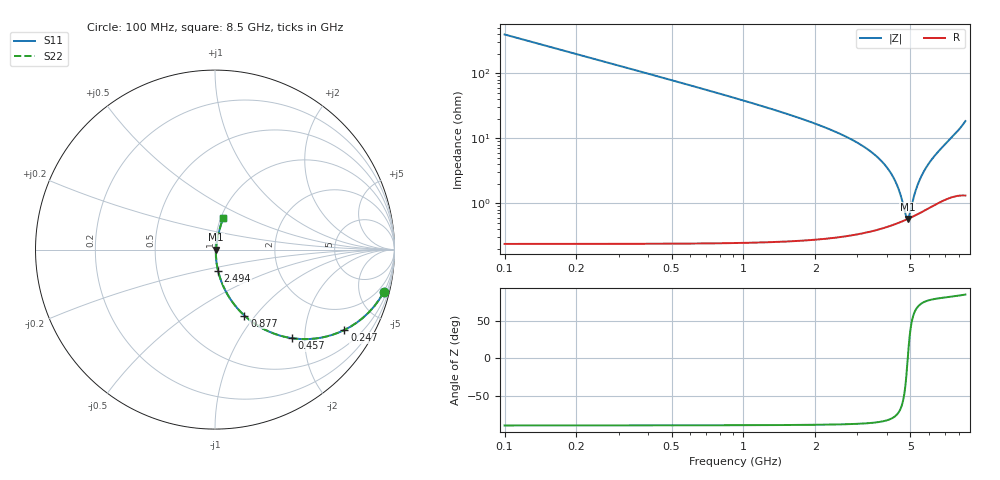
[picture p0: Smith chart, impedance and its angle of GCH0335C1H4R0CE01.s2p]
!Murata Part Number: GCH0335C1H4R0CE01
!These Parameters are Measured in Series Mode Connection
!Data Generated on Mar 13, 2026
!  o--ll--o
!Port1  Port2
!  o------o
!Operation Temp=25[degC], DC Bias Voltage=0[V]
!Freq. Start=100[MHz] Stop=9[GHz] 401[Steps]
# Hz S RI R 50
!Freq.(Hz) S11(Real) S11(Imag) S21(Real) S21(Imag) S12(Real) S12(Imag) S22(Real) S22(Imag)
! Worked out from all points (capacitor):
!   401 points, 100 MHz to 8.5 GHz, reference 50 ohm
!   read as one part in series: C = 4 pF near 142 MHz
!   lowest |Z| = 574 mohm at 4.867 GHz (marker M1)
!   series resonance near 4.875 GHz, so ESL is about 270 pH
!   S11 on the Smith chart (normalised r, x): 100 MHz: 1.00, -7.95; 247 MHz: 1.00, -3.21; 457 MHz: 1.00, -1.73; 877 MHz: 1.00, -0.88; 2.494 GHz: 1.01, -0.24; 8.5 GHz: 1.03, +0.37
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1e8  0.9404 -0.2364  0.0596 0.2364  0.0596 0.2364  0.9404 -0.2364
1.84e8  0.8232 -0.381  0.1768 0.381  0.1768 0.381  0.8232 -0.381
2.47e8  0.7206 -0.448  0.2794 0.448  0.2794 0.448  0.7206 -0.448
3.31e8  0.5888 -0.4911  0.4112 0.4911  0.4112 0.4911  0.5888 -0.4911
4.57e8  0.4275 -0.4933  0.5725 0.4933  0.5725 0.4933  0.4275 -0.4933
6.46e8  0.2695 -0.4417  0.7305 0.4417  0.7305 0.4417  0.2695 -0.4417
8.77e8  0.1639 -0.3674  0.8361 0.3674  0.8361 0.3674  0.1639 -0.3674
1.507e9  0.0571 -0.2268  0.9429 0.2268  0.9429 0.2268  0.0571 -0.2268
2.494e9  0.0173 -0.1186  0.9827 0.1186  0.9827 0.1186  0.0173 -0.1186
2.914e9  0.0114 -0.0898  0.9886 0.0898  0.9886 0.0898  0.0114 -0.0898
3.754e9  0.00611 -0.0456  0.9939 0.0456  0.9939 0.0456  0.00611 -0.0456
4.3e9  0.00523 -0.0222  0.9948 0.0222  0.9948 0.0222  0.00523 -0.0222
4.531e9  0.00527 -0.013  0.9947 0.013  0.9947 0.013  0.00527 -0.013
4.804e9  0.00559 -0.00264  0.9944 0.00264  0.9944 0.00264  0.00559 -0.00264
4.867e9  0.0057 -0.000292  0.9943 0.000292  0.9943 0.000292  0.0057 -0.000292
4.951e9  0.00588 0.00282  0.9941 -0.00282  0.9941 -0.00282  0.00588 0.00282
5.14e9  0.00636 0.00973  0.9936 -0.00973  0.9936 -0.00973  0.00636 0.00973
5.308e9  0.00689 0.0158  0.9931 -0.0158  0.9931 -0.0158  0.00689 0.0158
5.707e9  0.00853 0.03  0.9915 -0.03  0.9915 -0.03  0.00853 0.03
6.274e9  0.0118 0.0504  0.9882 -0.0504  0.9882 -0.0504  0.0118 0.0504
7.114e9  0.0186 0.0835  0.9814 -0.0835  0.9814 -0.0835  0.0186 0.0835
8.5e9  0.0447 0.1739  0.9553 -0.1739  0.9553 -0.1739  0.0447 0.1739
